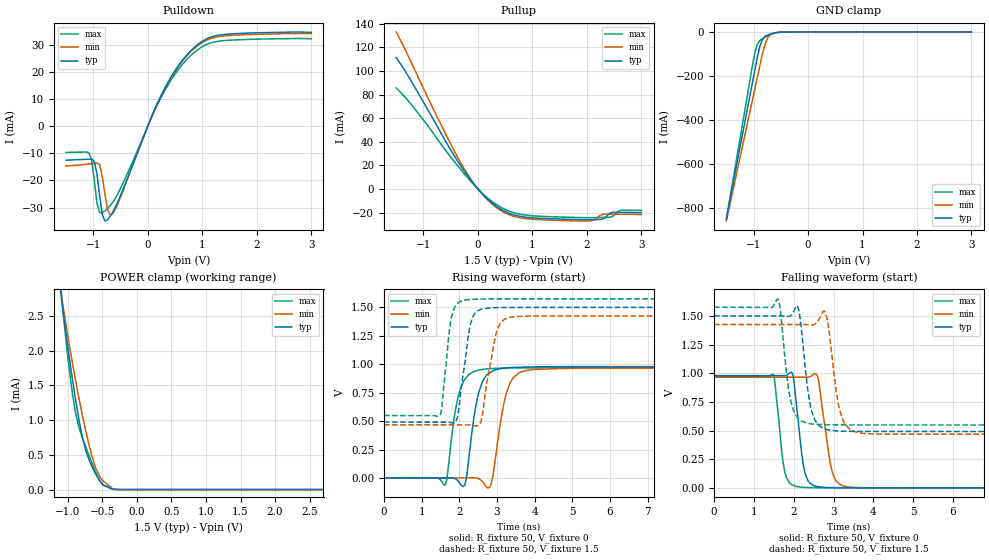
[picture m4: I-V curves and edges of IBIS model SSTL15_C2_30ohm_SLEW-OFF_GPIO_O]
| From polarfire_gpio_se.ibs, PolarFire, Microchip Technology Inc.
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|   Model SSTL15_C2_30ohm_SLEW-OFF_GPIO_O
[Model]   SSTL15_C2_30ohm_SLEW-OFF_GPIO_O
Model_type   Output
Polarity   Non-Inverting
Enable   Active-High
Vmeas =   0.75
Cref =   5p
Rref =   50
Vref =   0.75
|   typ   min   max
C_comp_pullup   2.605e-12   2.605e-12   2.76e-12
C_comp_pulldown  2.605e-12   2.605e-12   2.76e-12
[Temperature Range]  25C   100C   -40C
[Voltage Range]  1.5   1.425   1.575
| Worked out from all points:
|   slope of the pulldown table from 0 to 0.225 V, typ, clamps not added: 21.5 ohm
|   slope of the pullup table from 0 to 0.225 V, typ, clamps not added: 21.3 ohm
|   GND clamp passes 1 mA (typ) near -0.52 V on its own axis
|   POWER clamp passes 1 mA (typ) near -0.84 V on its own axis
|   rising waveform, R_fixture 50, V_fixture 0: 20-80 % time 288ps typ, 312ps min, 277ps max; typ from 0 V to 0.979 V
|   rising waveform, R_fixture 50, V_fixture 1.5: 20-80 % time 246ps typ, 295ps min, 195ps max; typ from 0.491 V to 1.5 V
|   falling waveform, R_fixture 50, V_fixture 0: 20-80 % time 195ps typ, 243ps min, 179ps max; typ from 0.979 V to 0 V
|   falling waveform, R_fixture 50, V_fixture 1.5: 20-80 % time 217ps typ, 240ps min, 211ps max; typ from 1.5 V to 0.491 V
[GND Clamp]
| Voltage   I(typ)   I(min)   I(max)
-1.5V     -849.7mA   -860.2mA   -853.5mA
-1.034V   -246.6mA   -324.3mA   -170.7mA
-984.4mV  -183.1mA   -267.7mA   -102.9mA
-935.2mV  -119.9mA   -211.2mA   -57.59mA
-885.9mV  -66.33mA   -154.7mA   -38.94mA
-836.7mV  -33.59mA   -99.09mA   -29.82mA
-787.5mV  -19.44mA   -53.53mA   -22.49mA
-738.3mV  -12.87mA   -24.95mA   -16.13mA
-689.1mV  -8.545mA   -11.57mA   -10.81mA
-590.6mV  -2.947mA   -3.067mA   -3.621mA
-393.7mV  -37.64uA   -63.17uA   -40.12uA
3V        0A         0A         0A
[POWER Clamp]
| Voltage   I(typ)   I(min)   I(max)
-1.5V     10.9mA     9.757mA    12.4mA
-1.23V    4.091mA    4.068mA    4.41mA
-1.083V   2.694mA    2.748mA    2.728mA
-984.4mV  1.956mA    2.133mA    1.792mA
-885.9mV  1.297mA    1.575mA    1.105mA
-787.5mV  756.7uA    1.072mA    746.1uA
-738.3mV  562.1uA    843.7uA    616.9uA
-590.6mV  217.4uA    298uA      241.2uA
-492.2mV  69.4uA     129.1uA    67.8uA
-344.5mV  1.546uA    8.832uA    4.546uA
-246.1mV  138.9nA    771.2nA    12.63nA
3V        0A         0A         0A
[Pullup]
| Voltage   I(typ)   I(min)   I(max)
-1.5V     111.3mA    133mA      85.62mA
-1.083V   80.2mA     93.42mA    63.35mA
-344.5mV  21.58mA    24.46mA    18.08mA
0V        -138.7nA   19.36uA    32.62uA
328.1mV   -14.33mA   -15.32mA   -12.86mA
656.2mV   -21.93mA   -23.17mA   -20.11mA
1.125V    -24.79mA   -25.99mA   -23.06mA
2.041V    -26.02mA   -27.05mA   -24.32mA
2.288V    -25.49mA   -21.55mA   -24.13mA
2.386V    -21.96mA   -21.3mA    -24.02mA
2.632V    -19.82mA   -21.45mA   -17.97mA
3V        -20mA      -21.64mA   -18.12mA
[Pulldown]
| Voltage   I(typ)   I(min)   I(max)
-1.5V     -12.55mA   -14.66mA   -9.693mA
-1.083V   -12.17mA   -13.94mA   -9.764mA
-984.4mV  -12.87mA   -13.68mA   -19.4mA
-935.2mV  -17.31mA   -13.54mA   -28.18mA
-885.9mV  -25.24mA   -14.07mA   -31.84mA
-836.7mV  -32.49mA   -18.41mA   -31.87mA
-738.3mV  -34.48mA   -30.75mA   -30.34mA
-590.6mV  -29.58mA   -30.37mA   -26.38mA
281.2mV   12.77mA    12.6mA     12.01mA
843.8mV   28.83mA    28.43mA    27mA
1.359V    33.68mA    33.12mA    31.41mA
3V        34.57mA    34.07mA    32.17mA
[Ramp]
dV/dt_r   0.587499/0.288311n  0.579688/0.311592n  0.581318/0.277044n
dV/dt_f   0.605181/0.217442n  0.574705/0.240398n  0.615737/0.210859n
R_load = 50
[Rising Waveform]
R_fixture = 50
V_fixture = 0
V_fixture_min = 0
V_fixture_max = 0
| Time   V(typ)   V(min)   V(max)
0s        10.75nV    15.04nV    15nV
1.617ns   731.1uV    401.7uV    -60.62mV
1.935ns   -15.91mV   480.7uV    667.8mV
2.12ns    -73.26mV   526.6uV    856mV
2.177ns   -18.76mV   540.8uV    879.8mV
2.507ns   741.8mV    -6.53mV    948.1mV
2.842ns   931.7mV    -55.24mV   962.1mV
3.244ns   966.8mV    740.2mV    967.8mV
3.6ns     973.9mV    927.8mV    968.2mV
10ns      979.2mV    966.1mV    968.9mV
[Rising Waveform]
R_fixture = 50
V_fixture = 1.5
V_fixture_min = 1.425
V_fixture_max = 1.575
| Time   V(typ)   V(min)   V(max)
0s        491.4mV    467.2mV    548.8mV
1.481ns   490.6mV    467mV      549.8mV
1.793ns   485.6mV    467mV      1.417V
1.944ns   528.5mV    467mV      1.53V
2.062ns   822.7mV    466.9mV    1.557V
2.379ns   1.43V      460mV      1.571V
2.578ns   1.483V     499.9mV    1.574V
2.974ns   1.498V     1.266V     1.575V
3.261ns   1.499V     1.405V     1.575V
10ns      1.5V       1.425V     1.575V
[Falling Waveform]
R_fixture = 50
V_fixture = 0
V_fixture_min = 0
V_fixture_max = 0
| Time   V(typ)   V(min)   V(max)
0s        979.2mV    966.1mV    968.9mV
1.491ns   978.5mV    965.5mV    985.8mV
1.778ns   978.1mV    965.4mV    136mV
1.976ns   989mV      965.3mV    23.96mV
2.079ns   691.8mV    965.3mV    10.99mV
2.362ns   60.19mV    965.7mV    2.796mV
2.608ns   10.46mV    964.4mV    941.1uV
2.957ns   1.847mV    154.6mV    38.55uV
3.221ns   564uV      19.52mV    37.14uV
10ns      -434.7nV   1.927uV    839.8nV
[Falling Waveform]
R_fixture = 50
V_fixture = 1.5
V_fixture_min = 1.425
V_fixture_max = 1.575
| Time   V(typ)   V(min)   V(max)
0s        1.5V       1.425V     1.575V
1.616ns   1.499V     1.425V     1.641V
1.868ns   1.495V     1.425V     867.6mV
2.1ns     1.58V      1.425V     610.3mV
2.361ns   840.7mV    1.423V     562mV
2.533ns   591.2mV    1.429V     554.9mV
2.8ns     512.1mV    1.525V     550.4mV
3.127ns   495.3mV    722.2mV    549.5mV
3.504ns   492.6mV    493.8mV    548.8mV
10ns      491.4mV    467.2mV    548.8mV
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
